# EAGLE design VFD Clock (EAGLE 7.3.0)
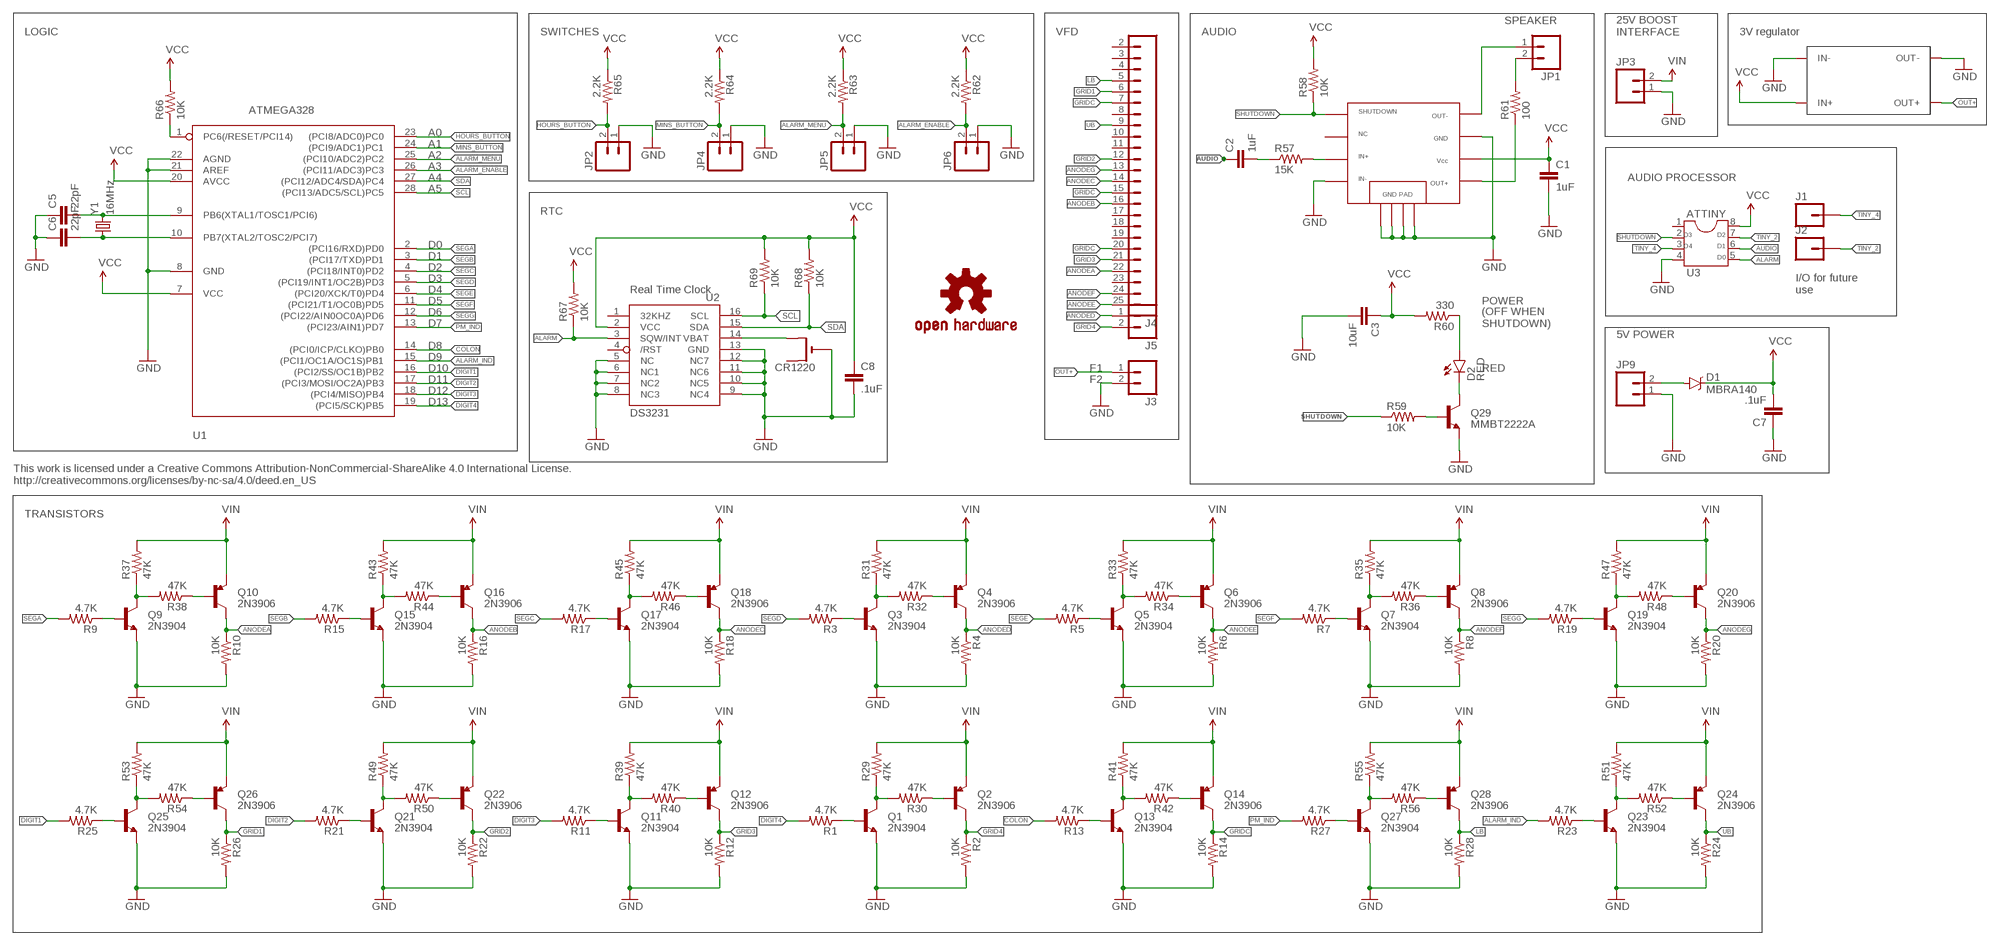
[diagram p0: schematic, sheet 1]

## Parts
ATTINY  U3  DIL8  [DIL08]
C1  1uF  CAPEZ  [CAP-PTH-SMALLEZ]
C2  1uF  CAPEZ  [CAP-PTH-SMALLEZ]
C3  10uF  CAPEZ  [CAP-PTH-SMALLEZ]
C5  22pF  CAPEZ  [CAP-PTH-SMALLEZ]
C6  22pF  CAPEZ  [CAP-PTH-SMALLEZ]
C7  .1uF  CAPEZ  [CAP-PTH-SMALLEZ]
C8  .1uF  CAPEZ  [CAP-PTH-SMALLEZ]
CR1220  CR1220SMT  [CR1220-SMD]
D1  MBRA140  [SMA-DIODE]
D2  RED  LED3MM  [LED3MM]
J1  M01PTH  [1X01]
J2  M01PTH  [1X01]
J3  M02PTH  [1X02]
J4  M24  [1X24]
J5  M02PTH  [1X02]
JP1  M02PTH  [1X02]
JP2  M02PTH  [1X02]
JP3  M02PTH  [1X02]
JP4  M02PTH  [1X02]
JP5  M02PTH  [1X02]
JP6  M02PTH  [1X02]
JP9  M02PTH  [1X02]
Q1  2N3904  TRANSISTOR_NPNTO-92-AMMO  [TO-92-AMMO]
Q2  2N3906  TRANSISTOR_PNPEBC  [TO-92-AMMO]
Q3  2N3904  TRANSISTOR_NPNTO-92-AMMO  [TO-92-AMMO]
Q4  2N3906  TRANSISTOR_PNPEBC  [TO-92-AMMO]
Q5  2N3904  TRANSISTOR_NPNTO-92-AMMO  [TO-92-AMMO]
Q6  2N3906  TRANSISTOR_PNPEBC  [TO-92-AMMO]
Q7  2N3904  TRANSISTOR_NPNTO-92-AMMO  [TO-92-AMMO]
Q8  2N3906  TRANSISTOR_PNPEBC  [TO-92-AMMO]
Q9  2N3904  TRANSISTOR_NPNTO-92-AMMO  [TO-92-AMMO]
Q10  2N3906  TRANSISTOR_PNPEBC  [TO-92-AMMO]
Q11  2N3904  TRANSISTOR_NPNTO-92-AMMO  [TO-92-AMMO]
Q12  2N3906  TRANSISTOR_PNPEBC  [TO-92-AMMO]
Q13  2N3904  TRANSISTOR_NPNTO-92-AMMO  [TO-92-AMMO]
Q14  2N3906  TRANSISTOR_PNPEBC  [TO-92-AMMO]
Q15  2N3904  TRANSISTOR_NPNTO-92-AMMO  [TO-92-AMMO]
Q16  2N3906  TRANSISTOR_PNPEBC  [TO-92-AMMO]
Q17  2N3904  TRANSISTOR_NPNTO-92-AMMO  [TO-92-AMMO]
Q18  2N3906  TRANSISTOR_PNPEBC  [TO-92-AMMO]
Q19  2N3904  TRANSISTOR_NPNTO-92-AMMO  [TO-92-AMMO]
Q20  2N3906  TRANSISTOR_PNPEBC  [TO-92-AMMO]
Q21  2N3904  TRANSISTOR_NPNTO-92-AMMO  [TO-92-AMMO]
Q22  2N3906  TRANSISTOR_PNPEBC  [TO-92-AMMO]
Q23  2N3904  TRANSISTOR_NPNTO-92-AMMO  [TO-92-AMMO]
Q24  2N3906  TRANSISTOR_PNPEBC  [TO-92-AMMO]
Q25  2N3904  TRANSISTOR_NPNTO-92-AMMO  [TO-92-AMMO]
Q26  2N3906  TRANSISTOR_PNPEBC  [TO-92-AMMO]
Q27  2N3904  TRANSISTOR_NPNTO-92-AMMO  [TO-92-AMMO]
Q28  2N3906  TRANSISTOR_PNPEBC  [TO-92-AMMO]
Q29  MMBT2222A  TRANSISTOR_NPNSOT23-3  [SOT23-3]
R1  4.7K  RESISTORPTH-1/4W-VERT  [AXIAL-0.1]
R2  10K  RESISTORPTH-1/4W-VERT  [AXIAL-0.1]
R3  4.7K  RESISTORPTH-1/4W-VERT  [AXIAL-0.1]
R4  10K  RESISTORPTH-1/4W-VERT  [AXIAL-0.1]
R5  4.7K  RESISTORPTH-1/4W-VERT  [AXIAL-0.1]
R6  10K  RESISTORPTH-1/4W-VERT  [AXIAL-0.1]
R7  4.7K  RESISTORPTH-1/4W-VERT  [AXIAL-0.1]
R8  10K  RESISTORPTH-1/4W-VERT  [AXIAL-0.1]
R9  4.7K  RESISTORPTH-1/4W-VERT  [AXIAL-0.1]
R10  10K  RESISTORPTH-1/4W-VERT  [AXIAL-0.1]
R11  4.7K  RESISTORPTH-1/4W-VERT  [AXIAL-0.1]
R12  10K  RESISTORPTH-1/4W-VERT  [AXIAL-0.1]
R13  4.7K  RESISTORPTH-1/4W-VERT  [AXIAL-0.1]
R14  10K  RESISTORPTH-1/4W-VERT  [AXIAL-0.1]
R15  4.7K  RESISTORPTH-1/4W-VERT  [AXIAL-0.1]
R16  10K  RESISTORPTH-1/4W-VERT  [AXIAL-0.1]
R17  4.7K  RESISTORPTH-1/4W-VERT  [AXIAL-0.1]
R18  10K  RESISTORPTH-1/4W-VERT  [AXIAL-0.1]
R19  4.7K  RESISTORPTH-1/4W-VERT  [AXIAL-0.1]
R20  10K  RESISTORPTH-1/4W-VERT  [AXIAL-0.1]
R21  4.7K  RESISTORPTH-1/4W-VERT  [AXIAL-0.1]
R22  10K  RESISTORPTH-1/4W-VERT  [AXIAL-0.1]
R23  4.7K  RESISTORPTH-1/4W-VERT  [AXIAL-0.1]
R24  10K  RESISTORPTH-1/4W-VERT  [AXIAL-0.1]
R25  4.7K  RESISTORPTH-1/4W-VERT  [AXIAL-0.1]
R26  10K  RESISTORPTH-1/4W-VERT  [AXIAL-0.1]
R27  4.7K  RESISTORPTH-1/4W-VERT  [AXIAL-0.1]
R28  10K  RESISTORPTH-1/4W-VERT  [AXIAL-0.1]
R29  47K  RESISTORPTH-1/4W-VERT  [AXIAL-0.1]
R30  47K  RESISTORPTH-1/4W-VERT  [AXIAL-0.1]
R31  47K  RESISTORPTH-1/4W-VERT  [AXIAL-0.1]
R32  47K  RESISTORPTH-1/4W-VERT  [AXIAL-0.1]
R33  47K  RESISTORPTH-1/4W-VERT  [AXIAL-0.1]
R34  47K  RESISTORPTH-1/4W-VERT  [AXIAL-0.1]
R35  47K  RESISTORPTH-1/4W-VERT  [AXIAL-0.1]
R36  47K  RESISTORPTH-1/4W-VERT  [AXIAL-0.1]
R37  47K  RESISTORPTH-1/4W-VERT  [AXIAL-0.1]
R38  47K  RESISTORPTH-1/4W-VERT  [AXIAL-0.1]
R39  47K  RESISTORPTH-1/4W-VERT  [AXIAL-0.1]
R40  47K  RESISTORPTH-1/4W-VERT  [AXIAL-0.1]
R41  47K  RESISTORPTH-1/4W-VERT  [AXIAL-0.1]
R42  47K  RESISTORPTH-1/4W-VERT  [AXIAL-0.1]
R43  47K  RESISTORPTH-1/4W-VERT  [AXIAL-0.1]
R44  47K  RESISTORPTH-1/4W-VERT  [AXIAL-0.1]
R45  47K  RESISTORPTH-1/4W-VERT  [AXIAL-0.1]
R46  47K  RESISTORPTH-1/4W-VERT  [AXIAL-0.1]
R47  47K  RESISTORPTH-1/4W-VERT  [AXIAL-0.1]
R48  47K  RESISTORPTH-1/4W-VERT  [AXIAL-0.1]
R49  47K  RESISTORPTH-1/4W-VERT  [AXIAL-0.1]
R50  47K  RESISTORPTH-1/4W-VERT  [AXIAL-0.1]
R51  47K  RESISTORPTH-1/4W-VERT  [AXIAL-0.1]
R52  47K  RESISTORPTH-1/4W-VERT  [AXIAL-0.1]
R53  47K  RESISTORPTH-1/4W-VERT  [AXIAL-0.1]
R54  47K  RESISTORPTH-1/4W-VERT  [AXIAL-0.1]
R55  47K  RESISTORPTH-1/4W-VERT  [AXIAL-0.1]
R56  47K  RESISTORPTH-1/4W-VERT  [AXIAL-0.1]
R57  15K  RESISTORPTH-1/4W-VERT  [AXIAL-0.1]
R58  10K  RESISTORPTH-1/4W-VERT  [AXIAL-0.1]
R59  10K  RESISTORPTH-1/4W-VERT  [AXIAL-0.1]
R60  330  RESISTORPTH-1/4W-VERT  [AXIAL-0.1]
R61  100  RESISTORPTH-1/4W-VERT  [AXIAL-0.1]
R62  2.2K  RESISTORPTH-1/4W-VERT  [AXIAL-0.1]
R63  2.2K  RESISTORPTH-1/4W-VERT  [AXIAL-0.1]
R64  2.2K  RESISTORPTH-1/4W-VERT  [AXIAL-0.1]
R65  2.2K  RESISTORPTH-1/4W-VERT  [AXIAL-0.1]
R66  10K  RESISTORPTH-1/4W-VERT  [AXIAL-0.1]
R67  10K  RESISTORPTH-1/4W-VERT  [AXIAL-0.1]
R68  10K  RESISTORPTH-1/4W-VERT  [AXIAL-0.1]
R69  10K  RESISTORPTH-1/4W-VERT  [AXIAL-0.1]
U1  ATMEGA328  ATMEGA168PROUND  [DIL28-3-ROUND]
U2  DS3231  DS3231/SO  [SO16W]
U3  TPA2005  [MSOP8]
U$7  OSHW-LOGOS  [OSHW-LOGO-S]
U$10  DCTODC  [DCTODC]
Y1  16MHz  CRYSTALHC49US  [HC49US]

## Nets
ALARM: ATTINY.5 R67.P$1 U2.3(SQW/INT)
ALARM_ENABLE: JP6.2 R62.P$2 U1.26((PCI11/ADC3)PC3)
ALARM_IND: R23.P$2 U1.15((PCI1/OC1A/OC1S)PB1)
ALARM_MENU: JP5.2 R63.P$2 U1.25((PCI10/ADC2)PC2)
ANODEA: J4.22 Q10.3(C) R10.P$1
ANODEB: J4.16 Q16.3(C) R16.P$1
ANODEC: J4.14 Q18.3(C) R18.P$1
ANODED: J5.1 Q4.3(C) R4.P$1
ANODEE: J4.25 Q6.3(C) R6.P$1
ANODEF: J4.24 Q8.3(C) R8.P$1
ANODEG: J4.13 Q20.3(C) R20.P$1
AUDIO: ATTINY.6 C2.1
COLON: R13.P$2 U1.14((PCI0/ICP/CLKO)PB0)
D: Q9.3(C) R37.P$1 R38.P$2
D1: Q15.3(C) R43.P$1 R44.P$2
D2: Q17.3(C) R45.P$1 R46.P$2
D3: Q3.3(C) R31.P$1 R32.P$2
D4: Q5.3(C) R33.P$1 R34.P$2
D5: Q7.3(C) R35.P$1 R36.P$2
D6: Q19.3(C) R47.P$1 R48.P$2
D7: Q25.3(C) R53.P$1 R54.P$2
D8: Q21.3(C) R49.P$1 R50.P$2
D9: Q11.3(C) R39.P$1 R40.P$2
D10: Q1.3(C) R29.P$1 R30.P$2
D11: Q13.3(C) R41.P$1 R42.P$2
D12: Q27.3(C) R55.P$1 R56.P$2
D13: Q23.3(C) R51.P$1 R52.P$2
DIGIT1: R25.P$2 U1.16((PCI2/SS/OC1B)PB2)
DIGIT2: R21.P$2 U1.17((PCI3/MOSI/OC2A)PB3)
DIGIT3: R11.P$2 U1.18((PCI4/MISO)PB4)
DIGIT4: R1.P$2 U1.19((PCI5/SCK)PB5)
GND: ATTINY.4 C1.2 C3.2 C5.1 C6.1 C7.1 C8.2 CR1220.- J3.2 JP2.1 JP3.1 JP4.1 JP5.1 JP6.1 JP9.1 Q1.1(E) Q3.1(E) Q5.1(E) Q7.1(E) Q9.1(E) Q11.1(E) Q13.1(E) Q15.1(E) Q17.1(E) Q19.1(E) Q21.1(E) Q23.1(E) Q25.1(E) Q27.1(E) Q29.2(E) R2.P$2 R4.P$2 R6.P$2 R8.P$2 R10.P$2 R12.P$2 R14.P$2 R16.P$2 R18.P$2 R20.P$2 R22.P$2 R24.P$2 R26.P$2 R28.P$2 U1.8(GND) U1.21(AREF) U1.22(AGND) U2.5(NC) U2.6(NC1) U2.7(NC2) U2.8(NC3) U2.9(NC4) U2.10(NC5) U2.11(NC6) U2.12(NC7) U2.13(GND) U3.4 U3.7 U3.A U3.B U3.C U3.D U$10.IN- U$10.OUT-
GRID1: J4.6 Q26.3(C) R26.P$1
GRID2: J4.12 Q22.3(C) R22.P$1
GRID3: J4.21 Q12.3(C) R12.P$1
GRID4: J5.2 Q2.3(C) R2.P$1
GRIDC: J4.7 J4.15 J4.20 Q14.3(C) R14.P$1
HOURS_BUTTON: JP2.2 R65.P$2 U1.23((PCI8/ADC0)PC0)
IN+AMP: R57.P$2 U3.3
LB: J4.5 Q28.3(C) R28.P$1
MINS_BUTTON: JP4.2 R64.P$2 U1.24((PCI9/ADC1)PC1)
N$1: Q15.2(B) R15.P$1
N$2: Q16.2(B) R44.P$1
N$3: Q17.2(B) R17.P$1
N$4: Q18.2(B) R46.P$1
N$5: Q3.2(B) R3.P$1
N$6: Q4.2(B) R32.P$1
N$7: CR1220.+$2(+1) U2.14(VBAT)
N$8: Q5.2(B) R5.P$1
N$9: Q6.2(B) R34.P$1
N$10: Q9.2(B) R9.P$1
N$11: Q7.2(B) R7.P$1
N$12: Q8.2(B) R36.P$1
N$13: Q10.2(B) R38.P$1
N$14: Q19.2(B) R19.P$1
N$15: Q20.2(B) R48.P$1
N$16: Q25.2(B) R25.P$1
N$17: Q26.2(B) R54.P$1
N$18: Q21.2(B) R21.P$1
N$19: Q22.2(B) R50.P$1
N$20: Q11.2(B) R11.P$1
N$21: Q12.2(B) R40.P$1
N$22: Q1.2(B) R1.P$1
N$23: Q2.2(B) R30.P$1
N$24: Q13.2(B) R13.P$1
N$25: Q14.2(B) R42.P$1
N$26: Q27.2(B) R27.P$1
N$27: Q28.2(B) R56.P$1
N$28: JP1.2 R61.P$2
N$29: D2.A R60.P$1
N$30: Q23.2(B) R23.P$1
N$31: Q29.1(B) R59.P$2
N$32: Q24.2(B) R52.P$1
N$33: D2.K(C) Q29.3(C)
N$34: C2.2 R57.P$1
N$35: JP1.1 U3.8
N$36: R61.P$1 U3.5
N$37: C5.2 U1.9(PB6(XTAL1/TOSC1/PCI6)) Y1.2
N$38: C6.2 U1.10(PB7(XTAL2/TOSC2/PCI7)) Y1.1
N$39: D1.A JP9.2
OUT+: J3.1 U$10.OUT+
PM_IND: R27.P$2 U1.13((PCI23/AIN1)PD7)
RESET: R66.P$1 U1.1(PC6(/RESET/PCI14))
SCL: R69.P$1 U1.28((PCI13/ADC5/SCL)PC5) U2.16(SCL)
SDA: R68.P$1 U1.27((PCI12/ADC4/SDA)PC4) U2.15(SDA)
SEGA: R9.P$2 U1.2((PCI16/RXD)PD0)
SEGB: R15.P$2 U1.3((PCI17/TXD)PD1)
SEGC: R17.P$2 U1.4((PCI18/INT0)PD2)
SEGD: R3.P$2 U1.5((PCI19/INT1/OC2B)PD3)
SEGE: R5.P$2 U1.6((PCI20/XCK/T0)PD4)
SEGF: R7.P$2 U1.11((PCI21/T1/OC0B)PD5)
SEGG: R19.P$2 U1.12((PCI22/AIN0OC0A)PD6)
SHUTDOWN: ATTINY.2 R58.P$1 R59.P$1 U3.1
TINY_2: ATTINY.7 J2.1
TINY_4: ATTINY.3 J1.1
UB: J4.9 Q24.3(C) R24.P$1
VCC: ATTINY.8 C1.1 C3.1 C7.2 C8.1 D1.C R58.P$2 R60.P$2 R62.P$1 R63.P$1 R64.P$1 R65.P$1 R66.P$2 R67.P$2 R68.P$2 R69.P$2 U1.7(VCC) U1.20(AVCC) U2.2(VCC) U3.6 U$10.IN+
VIN: JP3.2 Q2.1(E) Q4.1(E) Q6.1(E) Q8.1(E) Q10.1(E) Q12.1(E) Q14.1(E) Q16.1(E) Q18.1(E) Q20.1(E) Q22.1(E) Q24.1(E) Q26.1(E) Q28.1(E) R29.P$2 R31.P$2 R33.P$2 R35.P$2 R37.P$2 R39.P$2 R41.P$2 R43.P$2 R45.P$2 R47.P$2 R49.P$2 R51.P$2 R53.P$2 R55.P$2
Unconnected: ATTINY.1 CR1220.+$1(+) J4.2 J4.3 J4.4 J4.8 J4.10 J4.11 J4.17 J4.18 J4.19 J4.23 U2.1(32KHZ) U2.4(/RST) U3.NC

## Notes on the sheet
- SPEAKER
- LOGIC | SWITCHES | VFD | AUDIO
- 25V BOOST
  INTERFACE
- 3V regulator
- A0
- A1
- A2
- A3
- A4 | AUDIO PROCESSOR
- A5
- RTC
- D3 | D2
- D0 | D4 | D1
- D1 | D0
- D2
- D3
- D4 | Real Time Clock
- I/O for future
  use
- D5 | POWER
- D6
- D7
- (OFF WHEN 
  SHUTDOWN)
- 5V POWER
- D8
- D9
- D10 | F1 | RED
- D11 | F2
- D12
- D13
- This work is licensed under a Creative Commons Attribution-NonCommercial-ShareAlike 4.0 International License.
  http://creativecommons.org/licenses/by-nc-sa/4.0/deed.en_US
- TRANSISTORS

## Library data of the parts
ATTINY = ic-package:DIL8: Dual In Line / Socket
C1-C3 C5-C8 = SparkFun-Capacitors:CAP: Capacitor
CR1220 = adafruit:CR1220: CR1216/CR1220/CR1225 12mm 3V lithium coin cell Great for battery packup. Both SMT and THM holders. Note the THM package has the ground pads on both sides of the PCB so that the masks are the same - this reduces the cost
D1 = SparkFun-DiscreteSemi:MBRA140: 40V, 1A Schottky rectifier; PROD_ID: DIO-08053
D2 = SparkFun-LED:LED: LEDs; PROD_ID: DIO-08794
J1 J2 = SparkFun-Connectors:M01: Header 1
J3 J5 = SparkFun-Connectors:M02: Standard 2-pin 0.1" header. Use with
J4 = SparkFun-Connectors:M24: 1x24 .1" header
JP1-JP6 JP9 = SparkFun:M02: Header 2
Q1 Q3 Q5 Q7 Q9 Q11 Q13 Q15 Q17 Q19 Q21 Q23 Q25 Q27 = SparkFun-DiscreteSemi:TRANSISTOR_NPN: Generic NPN BJT MMBT2222A - TRANS-08049 (SOT-23, 1A 40V) MPSA42 - TRANS-09116 (SOT-23, 500mA 300V) MMBT5088LT1G - TRANS-11160 (SOT-23, 50 mA 30V)
Q2 Q4 Q6 Q8 Q10 Q12 Q14 Q16 Q18 Q20 Q22 Q24 Q26 Q28 = SparkFun-DiscreteSemi:TRANSISTOR_PNP: Generic PNP BJT Double check pinouts against datasheets- not all devices are the same! MMBT3906 - 40V 200mA SOT-23 (TRANS-08052) MMBT4403 - 40V 600mA SOT-23 (TRANS-09245)
Q29 = SparkFun:TRANSISTOR_NPN: Transistor NPN BJT configuration in SOT23 package. MMBT2222 is the common NPN we use. Double check BCE configuration again layout.
R1-R69 = SparkFun-Resistors:RESISTOR: Resistor
U1 = adafruit:ATMEGA168*P: MICROCONTROLLER 16 kBytes FLASH 1 kBytes SRAM 512 Bytes EEPROM USART 8-channel 10 bit ADC
U2 = adafruit:DS3231
U3 = TPA2005:TPA2005
U$7 = SparkFun:OSHW-LOGO: Open Source Hardware Logo This logo indicates the piece of hardware it is found on incorporates a OSHW license and/or adheres to the definition of open source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
U$10 = DC to DC:DCTODC
Y1 = SparkFun-FreqCtrl:CRYSTAL: Various standard crystals. Proven footprints.

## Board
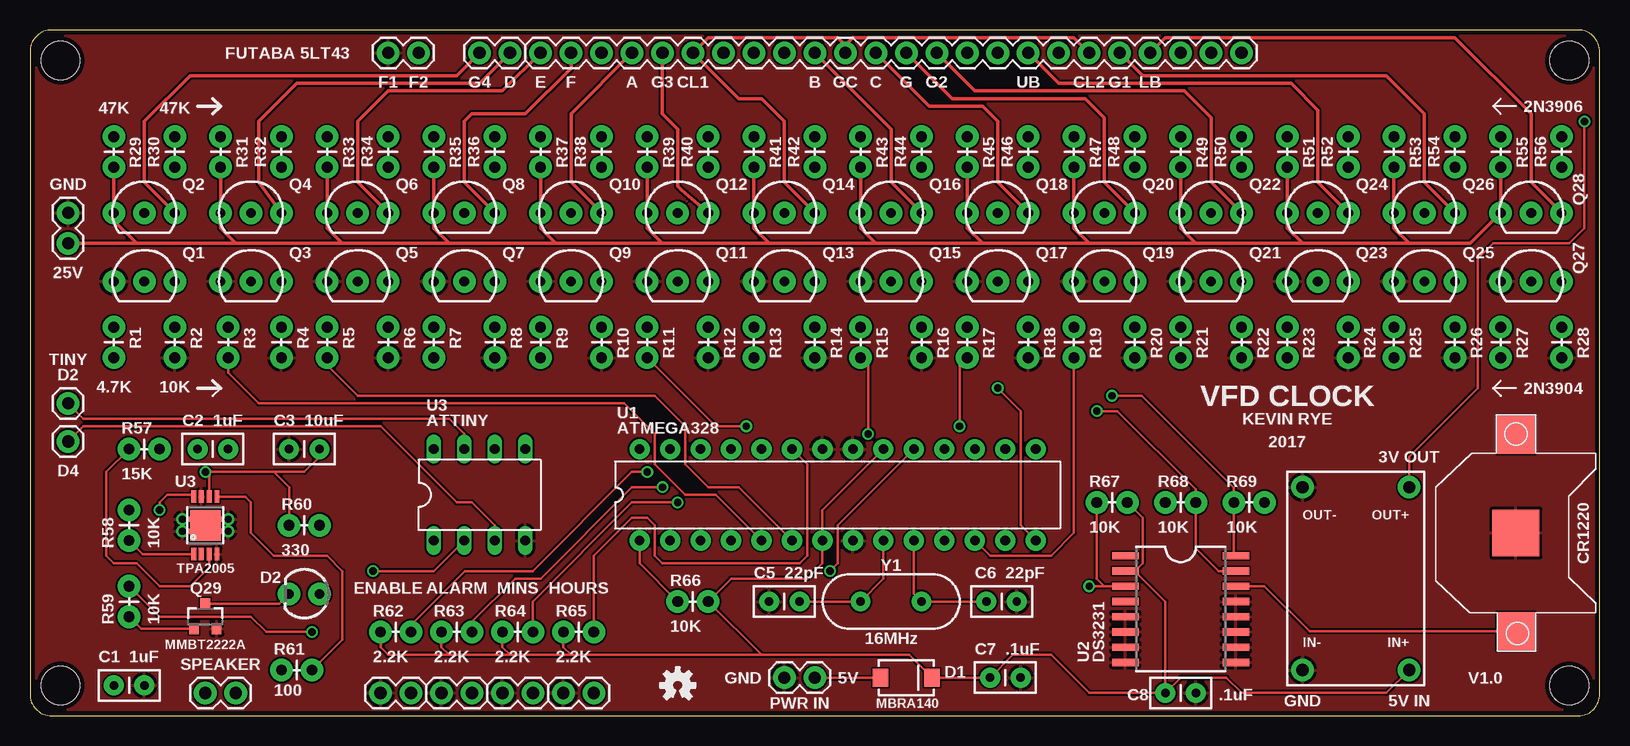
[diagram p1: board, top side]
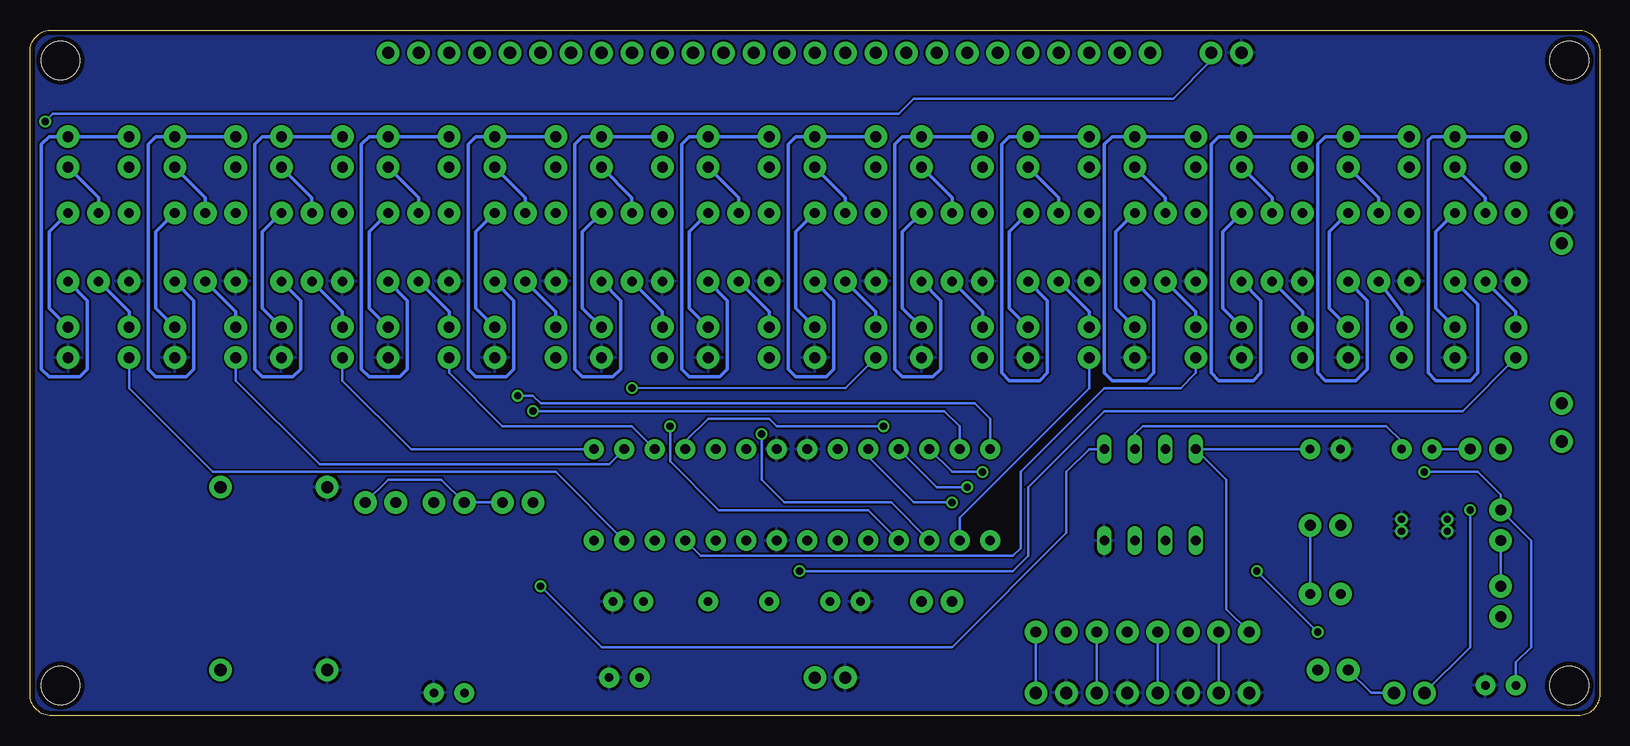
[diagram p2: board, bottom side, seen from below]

Size 130.81 x 57.15 mm. Coordinates in mm from the lower left corner, seen from the top.
Outline: 0,55.35 0,1.8 arc90 1.8,0 129.01,0 arc90 130.81,1.8 130.81,55.35 arc90 129.01,57.15 1.8,57.15 arc90 0,55.35
Copper layers (1*16): Top 0.0356mm / dielectric 1.5011mm / Bottom 0.0356mm
Design rules "oshpark-2layer": minimum track width 6mil, minimum drill 13mil, track to track 6mil, track to pad 6mil, pad to pad 6mil, via to via 6mil, smd to smd 6mil, copper to edge 15mil, drill to drill 6mil, minimum pad ring 7mil, minimum via ring 7mil, stop-mask expansion 2.5mil, vias tented up to drill 0mil, thermal gap 10mil
Holes 3.2 mm at 2.54,54.61 128.27,54.61 128.27,2.54 2.54,2.54

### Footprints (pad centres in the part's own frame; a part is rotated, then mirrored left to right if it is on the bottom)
DIL08 = drill 0.813 long: 1 -3.81,-3.81; 2 -1.27,-3.81; 3 1.27,-3.81; 4 3.81,-3.81; 5 3.81,3.81; 6 1.27,3.81; 7 -1.27,3.81; 8 -3.81,3.81
CAP-PTH-SMALLEZ = drill 0.7 pad 1.651: 1 0,0; 2 2.54,0
CR1220-SMD = smd 3.2 x 3.2: +$1 -8.2,0; +$2 8.2,0 | smd 3.9 x 3.9: - 0,0
SMA-DIODE = smd 1.27 x 1.47: A -2.15,0; C 2.15,0
LED3MM = drill 0.813 pad 1.88: A -1.27,0; K 1.27,0
1X01 = drill 1.016 pad 1.88: 1 0,0
1X02 = drill 1.016 pad 1.88: 1 0,0; 2 2.54,0
1X24 = drill 1.016 pad 1.88: 2 -26.67,0; 3 -24.13,0; 4 -21.59,0; 5 -19.05,0; 6 -16.51,0; 7 -13.97,0; 8 -11.43,0; 9 -8.89,0; 10 -6.35,0; 11 -3.81,0; 12 -1.27,0; 13 1.27,0; 14 3.81,0; 15 6.35,0; 16 8.89,0; 17 11.43,0; 18 13.97,0; 19 16.51,0; 20 19.05,0; 21 21.59,0; 22 24.13,0; 23 26.67,0; 24 29.21,0; 25 31.75,0
TO-92-AMMO = drill 0.813 pad 1.88: 1 -2.54,0; 2 0,0; 3 2.54,0
SOT23-3 = smd 0.8 x 0.9: 1 -0.95,-1; 2 0.95,-1; 3 0,1.1
AXIAL-0.1 = drill 0.9 pad 1.88: P$1 0,0; P$2 2.54,0
DIL28-3-ROUND = drill 0.813 pad 1.676: 1 -16.51,-3.81; 2 -13.97,-3.81; 3 -11.43,-3.81; 4 -8.89,-3.81; 5 -6.35,-3.81; 6 -3.81,-3.81; 7 -1.27,-3.81; 8 1.27,-3.81; 9 3.81,-3.81; 10 6.35,-3.81; 11 8.89,-3.81; 12 11.43,-3.81; 13 13.97,-3.81; 14 16.51,-3.81; 15 16.51,3.81; 16 13.97,3.81; 17 11.43,3.81; 18 8.89,3.81; 19 6.35,3.81; 20 3.81,3.81; 21 1.27,3.81; 22 -1.27,3.81; 23 -3.81,3.81; 24 -6.35,3.81; 25 -8.89,3.81; 26 -11.43,3.81; 27 -13.97,3.81; 28 -16.51,3.81
SO16W = smd 0.6 x 2.2: 1 -4.445,-4.6; 2 -3.175,-4.6; 3 -1.905,-4.6; 4 -0.635,-4.6; 5 0.635,-4.6; 6 1.905,-4.6; 7 3.175,-4.6; 8 4.445,-4.6; 9 4.445,4.6; 10 3.175,4.6; 11 1.905,4.6; 12 0.635,4.6; 13 -0.635,4.6; 14 -1.905,4.6; 15 -3.175,4.6; 16 -4.445,4.6
MSOP8 = smd 0.41 x 1.02: 1 -0.975,-2.4; 3 0.325,-2.4; 4 0.975,-2.4; 5 0.975,2.4; 6 0.325,2.4; 7 -0.325,2.4; 8 -0.975,2.4; NC -0.325,-2.4 | smd 1.02 x 0.41: 2 -1.13,0.5; 9 -1.13,-0.5; 10 1.13,-0.5; 11 1.13,0.5 | drill 0.61 pad 1.016: A -1.9,-0.5; B 1.91,-0.5; C 1.91,0.5; D -1.9,0.5 | smd 2.54 x 1.27: GND 0,0.635; GND1 0,0.635; GND* 0,-0.635
DCTODC = drill 1.016 pad 1.88: IN+ 10.16,1.27; IN- 1.27,1.27; OUT+ 10.16,16.51; OUT- 1.27,16.51
HC49US = drill 0.7 pad 1.651: 1 -2.54,0; 2 2.54,0

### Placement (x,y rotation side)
ATTINY  37.47,18.41 0 top
C1  6.99,2.54 0 top
C2  16.51,22.23 180 top
C3  24.13,22.23 180 top
C5  61.59,9.53 0 top
C6  82.23,9.53 180 top
C7  82.55,3.18 180 top
C8  94.61,1.91 0 top
CR1220  123.82,15.24 270 top
D1  73.02,3.18 0 top
D2  22.86,10.16 180 top
J1  3.17,22.86 0 top
J2  3.17,26.04 0 top
J3  32.39,55.24 180 top
J4  74.3,55.24 180 top
J5  40.01,55.24 180 top
JP1  14.61,1.91 0 top
JP2  44.45,1.91 0 top
JP3  3.17,41.91 270 top
JP4  39.37,1.91 0 top
JP5  34.29,1.91 0 top
JP6  29.21,1.91 0 top
JP9  62.87,3.18 0 top
Q1  9.53,36.2 0 top
Q2  9.53,41.91 0 top
Q3  18.41,36.2 0 top
Q4  18.41,41.91 0 top
Q5  27.3,36.2 0 top
Q6  27.3,41.91 0 top
Q7  36.2,36.2 0 top
Q8  36.2,41.91 0 top
Q9  45.09,36.2 0 top
Q10  45.09,41.91 0 top
Q11  53.98,36.2 0 top
Q12  53.98,41.91 0 top
Q13  62.87,36.2 0 top
Q14  62.87,41.91 0 top
Q15  71.75,36.2 0 top
Q16  71.75,41.91 0 top
Q17  80.64,36.2 0 top
Q18  80.64,41.91 0 top
Q19  89.53,36.2 0 top
Q20  89.53,41.91 0 top
Q21  98.42,36.2 0 top
Q22  98.42,41.91 0 top
Q23  107.31,36.2 0 top
Q24  107.31,41.91 0 top
Q25  116.2,36.2 0 top
Q26  116.2,41.91 0 top
Q27  125.09,36.2 0 top
Q28  125.09,41.91 0 top
Q29  14.61,8.26 0 top
R1  6.99,32.38 270 top
R2  12.06,32.38 270 top
R3  16.51,32.38 270 top
R4  20.95,32.38 270 top
R5  24.76,32.38 270 top
R6  29.84,32.38 270 top
R7  33.66,32.38 270 top
R8  38.73,32.38 270 top
R9  42.55,32.38 270 top
R10  47.62,32.38 270 top
R11  51.44,32.38 270 top
R12  56.52,32.38 270 top
R13  60.33,32.38 270 top
R14  65.41,32.38 270 top
R15  69.21,32.38 270 top
R16  74.3,32.38 270 top
R17  78.1,32.38 270 top
R18  83.18,32.38 270 top
R19  86.99,32.38 270 top
R20  92.07,32.38 270 top
R21  95.88,32.38 270 top
R22  100.96,32.38 270 top
R23  104.77,32.38 270 top
R24  109.85,32.38 270 top
R25  113.66,32.38 270 top
R26  118.74,32.38 270 top
R27  122.55,32.38 270 top
R28  127.64,32.38 270 top
R29  6.99,48.26 270 top
R30  12.06,45.72 90 top
R31  15.88,48.26 270 top
R32  20.95,45.72 90 top
R33  24.76,48.26 270 top
R34  29.84,45.72 90 top
R35  33.66,48.26 270 top
R36  38.73,45.72 90 top
R37  42.55,48.26 270 top
R38  47.62,45.72 90 top
R39  51.44,48.26 270 top
R40  56.52,45.72 90 top
R41  60.33,48.26 270 top
R42  65.41,45.72 90 top
R43  69.21,48.26 270 top
R44  74.3,45.72 90 top
R45  78.1,48.26 270 top
R46  83.18,45.72 90 top
R47  86.99,48.26 270 top
R48  92.07,45.72 90 top
R49  95.88,48.26 270 top
R50  100.96,45.72 90 top
R51  104.77,48.26 270 top
R52  109.85,45.72 90 top
R53  113.66,48.26 270 top
R54  118.74,45.72 90 top
R55  122.55,48.26 270 top
R56  127.64,45.72 90 top
R57  10.79,22.23 180 top
R58  8.26,14.61 90 top
R59  8.26,10.8 270 top
R60  24.13,15.88 180 top
R61  23.49,3.81 180 top
R62  29.21,6.98 0 top
R63  34.29,6.98 0 top
R64  39.37,6.98 0 top
R65  44.45,6.98 0 top
R66  53.98,9.53 0 top
R67  88.9,17.78 0 top
R68  97.16,17.78 180 top
R69  100.33,17.78 0 top
U1  67.31,18.41 0 top
U2  95.88,8.89 270 top
U3  14.61,15.88 0 top
U$7  53.98,2.54 0 top
U$10  104.77,2.54 0 top
Y1  71.75,9.53 180 top

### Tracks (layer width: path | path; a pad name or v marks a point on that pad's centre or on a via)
ALARM  (via drill 0.61)
  Top 0.203: U2.3 89.53,10.8 | 89.53,10.8 88.9,11.43 R67.P$1 | v88.27,10.8 89.53,10.8
  Bottom 0.203: ATTINY.5 42.55,22.23 44.45,20.32 44.45,15.24 53.98,5.71 83.18,5.71 v88.27,10.8
ALARM_ENABLE  (via drill 0.61)
  Top 0.203: v51.44,20.32 50.16,20.32 41.91,12.07 36.24,12.07 31.75,7.57 R62.P$2
  Bottom 0.203: JP6.2 R62.P$2 | U1.26 53.98,20.32 v51.44,20.32
ALARM_IND
  Bottom 0.203: U1.15 99.06,22.23 104.77,27.94 R23.P$2
ALARM_MENU  (via drill 0.61)
  Top 0.203: v52.71,19.05 50.16,19.05 42.55,11.43 40.42,11.43 36.83,7.84 R63.P$2
  Bottom 0.203: JP5.2 R63.P$2 | U1.25 55.25,19.05 v52.71,19.05
ANODEA
  Top 0.305: Q10.3 45.09,44.45 45.09,50.16 J4.22
  Bottom 0.305: Q10.3 49.21,40.32 49.21,33.97 R10.P$1
ANODEB
  Top 0.305: Q16.3 71.75,44.45 71.75,48.9 J4.16
  Bottom 0.305: R16.P$1 75.88,33.97 75.88,40.32 Q16.3
ANODEC
  Top 0.305: Q18.3 80.64,44.45 80.64,49.53 79.38,50.8 74.93,50.8 J4.14
  Bottom 0.305: R18.P$1 84.77,33.97 84.77,40.32 Q18.3
ANODED
  Top 0.305: Q4.3 19.05,44.45 19.05,49.53 22.22,52.71 37.47,52.71 J5.1
  Bottom 0.305: R4.P$1 22.54,33.97 22.54,40.32 Q4.3
ANODEE
  Top 0.305: Q6.3 27.3,44.45 27.3,49.53 29.84,52.07 39.37,52.07 J4.25
  Bottom 0.305: R6.P$1 31.43,33.97 31.43,40.32 Q6.3
ANODEF
  Top 0.305: Q8.3 36.2,44.45 36.2,49.53 36.83,50.16 41.27,50.16 45.09,53.98 J4.24
  Bottom 0.305: R8.P$1 40.32,33.97 40.32,40.32 Q8.3
ANODEG
  Top 0.305: Q20.3 89.53,44.45 89.53,49.85 87.95,51.43 76.83,51.43 J4.13
  Bottom 0.305: R20.P$1 93.66,33.97 93.66,40.32 Q20.3
AUDIO
  Bottom 0.203: C2.1 16.51,22.86 17.78,24.13 38.1,24.13 38.73,23.49 ATTINY.6
COLON  (via drill 0.61)
  Top 0.203: U1.14 82.55,15.88 82.55,25.4 v80.64,27.3
  Bottom 0.178: 62.87,27.3 v80.64,27.3
  Bottom 0.203: R13.P$2 62.87,27.3
D
  Bottom 0.305: R37.P$1 R38.P$2 49.21,48.26 49.85,47.63 49.85,28.58 49.21,27.94 46.67,27.94 46.04,28.58 46.04,34.61 Q9.3
D1
  Bottom 0.305: R43.P$1 R44.P$2 75.88,48.26 76.52,47.63 76.52,28.89 75.88,28.26 73.34,28.26 72.71,28.89 72.71,34.61 Q15.3
D2
  Bottom 0.305: R45.P$1 R46.P$2 84.77,48.26 85.41,47.63 85.41,28.89 84.77,28.26 82.23,28.26 81.6,28.89 81.6,34.61 Q17.3
D3
  Bottom 0.305: R31.P$1 R32.P$2 22.86,48.26 23.49,47.63 23.49,28.58 22.86,27.94 20.32,27.94 19.37,28.89 19.37,34.61 Q3.3
D4
  Bottom 0.305: R33.P$1 R34.P$2 31.75,48.26 32.39,47.63 32.39,28.58 31.75,27.94 28.89,27.94 28.26,28.58 28.26,34.61 Q5.3
D5
  Bottom 0.305: R35.P$1 R36.P$2 40.64,48.26 41.27,47.63 41.27,28.58 40.64,27.94 37.78,27.94 37.15,28.58 37.15,34.61 Q7.3
D6
  Bottom 0.305: R47.P$1 R48.P$2 93.66,48.26 94.3,47.63 94.3,28.89 93.66,28.26 91.12,28.26 90.49,28.89 90.49,34.61 Q19.3
D7
  Bottom 0.305: R53.P$1 R54.P$2 120.33,48.26 120.97,47.63 120.97,28.89 120.33,28.26 117.79,28.26 117.16,28.89 117.16,34.61 Q25.3
D8
  Bottom 0.305: R49.P$1 R50.P$2 102.55,48.26 103.19,47.63 103.19,28.89 102.55,28.26 100.01,28.26 99.38,28.89 99.38,34.61 Q21.3
D9
  Bottom 0.305: R39.P$1 R40.P$2 58.1,48.26 58.74,47.63 58.74,28.89 58.1,28.26 55.56,28.26 54.93,28.89 54.93,34.61 Q11.3
D10
  Bottom 0.305: R29.P$1 R30.P$2 13.97,48.26 14.29,47.94 14.29,28.58 13.65,27.94 10.79,27.94 10.16,28.58 10.16,34.29 Q1.3
D11
  Bottom 0.305: R41.P$1 R42.P$2 66.99,48.26 67.63,47.63 67.63,28.89 66.99,28.26 64.45,28.26 63.82,28.89 63.82,34.61 Q13.3
D12
  Bottom 0.305: R55.P$1 R56.P$2 129.22,48.26 129.86,47.63 129.86,28.89 129.22,28.26 126.68,28.26 126.05,28.89 126.05,34.61 Q27.3
D13
  Bottom 0.305: R51.P$1 R52.P$2 111.44,48.26 112.08,47.63 112.08,28.89 111.44,28.26 108.9,28.26 108.27,28.89 108.27,34.61 Q23.3
DIGIT1
  Bottom 0.203: U1.16 82.55,20.95 106.68,20.95 113.66,27.94 R25.P$2
DIGIT2
  Bottom 0.203: R21.P$2 95.88,28.58 91.44,24.13 80.64,24.13 U1.17
DIGIT3  (via drill 0.61)
  Top 0.203: v59.69,24.13 57.15,24.13 R11.P$2
  Bottom 0.203: U1.18 76.2,22.86 74.3,24.77 69.21,24.77 68.58,24.13 v59.69,24.13
DIGIT4  (via drill 0.61)
  Top 0.203: v66.67,12.07 67.31,12.7 67.31,15.88 U1.19
  Bottom 0.203: R1.P$2 11.43,25.4 41.27,25.4 47.62,19.05 47.62,13.34 48.9,12.07 v66.67,12.07
GND
  pour Bottom: -0.64,57.79 131.45,57.79 131.45,-0.63 -0.64,-0.63
  pour Top: -1.27,58.42 132.4,58.42 132.4,-1.27 -1.27,-1.27
GRID1
  Top 0.305: Q26.3 116.2,44.45 116.2,50.16 113.03,53.34 92.71,53.34 J4.6
  Bottom 0.305: R26.P$1 120.33,33.97 120.33,40.32 Q26.3
GRID2
  Top 0.305: Q22.3 98.42,44.45 98.42,49.85 96.2,52.07 78.74,52.07 J4.12
  Bottom 0.305: R22.P$1 102.55,33.97 102.55,40.32 Q22.3
GRID3
  Top 0.305: Q12.3 54.29,43.81 53.98,44.13 53.98,48.9 52.71,50.16 J4.21
  Bottom 0.305: Q12.3 58.1,40.32 58.1,33.97 R12.P$1
GRID4
  Top 0.305: Q2.3 9.53,44.45 9.53,49.53 13.34,53.34 35.56,53.34 J5.2
  Bottom 0.305: R2.P$1 13.65,33.97 13.65,40.32 Q2.3
GRIDC
  Top 0.305: Q14.3 62.87,44.45 62.87,49.53 60.96,51.43 59.05,51.43 J4.20 56.52,56.52 67.31,56.52 67.94,55.88 | J4.15 67.94,55.88 | 67.94,55.88 68.58,56.52 86.99,56.52 J4.7
  Bottom 0.305: R14.P$1 66.99,33.97 66.99,40.32 Q14.3
HOURS_BUTTON
  Top 0.203: U1.23 64.77,20.95 64.77,13.34 64.13,12.7 52.71,12.7 52.07,13.34 52.07,15.88 51.44,16.51 50.16,16.51 46.99,13.34 R65.P$2
  Bottom 0.203: JP2.2 R65.P$2
IN+AMP
  Top 0.203: U3.3 14.93,12.39 13.34,10.8 10.79,10.8 8.89,12.7 6.99,12.7 6.35,13.34 6.35,20.32 R57.P$2
LB
  Top 0.305: Q28.3 125.09,44.45 125.09,50.16 118.74,56.52 94.61,56.52 J4.5
  Bottom 0.305: R28.P$1 129.22,33.97 129.22,40.32 Q28.3
MINS_BUTTON  (via drill 0.61)
  Top 0.203: v53.98,17.78 50.16,17.78 41.91,9.53 R64.P$2
  Bottom 0.203: JP4.2 R64.P$2 | U1.24 60.96,21.59 57.15,17.78 v53.98,17.78
N$1
  Bottom 0.305: R15.P$1 69.21,33.66 Q15.2
N$2
  Bottom 0.305: Q16.2 71.75,43.18 R44.P$1
N$3
  Bottom 0.305: R17.P$1 78.1,33.66 Q17.2
N$4
  Bottom 0.305: Q18.2 80.64,43.18 R46.P$1
N$5
  Bottom 0.305: R3.P$1 16.51,33.66 Q3.2
N$6
  Bottom 0.305: Q4.2 18.41,43.18 R32.P$1
N$7
  Top 0.203: CR1220.+$2 106.62,7.04 102.87,10.8 U2.14
N$8
  Bottom 0.305: R5.P$1 24.76,33.66 Q5.2
N$9
  Bottom 0.305: Q6.2 27.3,43.18 R34.P$1
N$10
  Bottom 0.305: R9.P$1 42.55,33.66 Q9.2
N$11
  Bottom 0.305: R7.P$1 33.66,33.66 Q7.2
N$12
  Bottom 0.305: Q8.2 36.2,43.18 R36.P$1
N$13
  Bottom 0.305: Q10.2 45.09,43.18 R38.P$1
N$14
  Bottom 0.305: R19.P$1 86.99,33.66 Q19.2
N$15
  Bottom 0.305: Q20.2 89.53,43.18 R48.P$1
N$16
  Bottom 0.305: R25.P$1 113.66,33.66 Q25.2
N$17
  Bottom 0.305: Q26.2 116.2,43.18 R54.P$1
N$18
  Bottom 0.305: R21.P$1 95.88,33.66 Q21.2
N$19
  Bottom 0.305: Q22.2 98.42,43.18 R50.P$1
N$20
  Bottom 0.305: R11.P$1 51.44,33.66 Q11.2
N$21
  Bottom 0.305: Q12.2 53.98,43.18 R40.P$1
N$22
  Bottom 0.305: R1.P$1 6.99,33.66 Q1.2
N$23
  Bottom 0.305: Q2.2 9.53,43.18 R30.P$1
N$24
  Bottom 0.305: R13.P$1 60.33,33.66 Q13.2
N$25
  Bottom 0.305: Q14.2 62.87,43.18 R42.P$1
N$26
  Bottom 0.305: R27.P$1 122.55,33.66 Q27.2
N$27
  Bottom 0.305: Q28.2 125.09,43.18 R56.P$1
N$28
  Bottom 0.203: JP1.2 19.05,1.91 R61.P$2
N$29
  Bottom 0.203: R60.P$1 D2.A
N$30
  Bottom 0.305: R23.P$1 104.77,33.66 Q23.2
N$31
  Top 0.203: Q29.1 9.26,7.26 R59.P$2
N$32
  Bottom 0.305: Q24.2 107.31,43.18 R52.P$1
N$33
  Top 0.203: Q29.3 20.79,9.36 D2.K
N$34
  Bottom 0.203: R57.P$1 C2.2
N$35  (via drill 0.61)
  Top 0.203: v10.79,17.15 10.79,17.78 11.43,18.41 13.49,18.41 U3.8
  Bottom 0.203: JP1.1 10.79,5.71 v10.79,17.15
N$36
  Top 0.203: U3.5 17.92,18.27 18.41,17.78 18.41,15.24 20.32,13.34 24.76,13.34 26.04,12.07 26.04,6.35 R61.P$1
N$37
  Top 0.203: C5.2 Y1.2 71.12,11.43 U1.9
N$38
  Top 0.203: C6.2 Y1.1 73.66,10.16 U1.10
N$39
  Top 0.203: JP9.2 D1.A
OUT+  (via drill 0.61)
  Top 0.203: v129.54,49.53 129.54,40.64 128.27,39.37 121.92,39.37 120.65,38.1 120.65,27.3 114.93,21.59 U$10.OUT+
  Bottom 0.203: J3.1 32.39,54.61 35.56,51.43 57.15,51.43 58.42,50.16 128.91,50.16 v129.54,49.53
PM_IND
  Bottom 0.203: U1.13 86.99,20.32 115.57,20.32 122.55,27.3 R27.P$2
RESET
  Top 0.203: R66.P$1 50.8,12.7 U1.1
SCL  (via drill 0.61)
  Top 0.203: U2.16 100.33,13.65 R69.P$1 100.33,19 92.66,26.67 v90.17,26.67
  Bottom 0.203: U1.28 50.8,24.77 52.07,26.04 88.27,26.04 88.9,26.67 v90.17,26.67
SDA  (via drill 0.61)
  Top 0.203: U2.15 99.06,12.07 97.16,13.97 R68.P$1 97.16,18.86 90.62,25.4 v88.9,25.4
  Bottom 0.203: U1.27 53.34,24.13 54.61,25.4 v88.9,25.4
SEGA
  Bottom 0.203: U1.2 53.34,16.51 42.55,27.3 R9.P$2
SEGB  (via drill 0.61)
  Top 0.203: R15.P$2 69.85,29.21 v69.85,23.49
  Bottom 0.203: v69.85,23.49 69.85,19.69 67.94,17.78 59.05,17.78 U1.3
SEGC  (via drill 0.61)
  Top 0.203: R17.P$2 77.47,29.21 v77.47,24.13
  Bottom 0.203: v77.47,24.13 77.47,21.21 73.4,17.15 60.96,17.15 U1.4
SEGD
  Top 0.203: R3.P$2 16.51,28.58 19.05,26.04 49.53,26.04 52.07,23.49 52.07,20.95 54.61,18.41 57.15,18.41 U1.5
SEGE
  Top 0.203: R5.P$2 24.76,29.21 27.3,26.67 52.07,26.67 54.61,24.13 54.61,20.95 56.52,19.05 59.05,19.05 U1.6
SEGF
  Bottom 0.203: R7.P$2 33.66,28.58 34.93,27.3 41.27,27.3 48.26,20.32 48.26,13.97 48.9,13.34 74.93,13.34 U1.11
SEGG
  Top 0.203: U1.12 80.01,13.34 85.09,13.34 86.99,15.24 R19.P$2
SHUTDOWN  (via drill 0.61)
  Top 0.203: U3.1 9.38,13.48 R58.P$1 | ATTINY.2 33.66,12.07 v28.57,12.07 | R59.P$1 10.79,8.26 18.41,8.26 19.68,6.98 v23.49,6.98
  Bottom 0.203: R58.P$1 R59.P$1 | v28.57,12.07 23.81,7.3 v23.49,6.98
TINY_2
  Top 0.203: ATTINY.7 36.2,23.49 34.93,24.77 4.45,24.77 J2.1
TINY_4
  Top 0.203: J1.1 4.45,24.13 29.21,24.13 35.56,17.78 36.83,17.78 38.73,15.88 ATTINY.3
UB
  Top 0.305: Q24.3 107.31,44.45 107.31,50.48 105.09,52.71 85.72,52.71 J4.9
  Bottom 0.305: R24.P$1 111.44,33.97 111.44,40.32 Q24.3
VCC  (via drill 0.61)
  Top 0.203: U1.20 66.04,17.15 U1.7 66.04,12.7 64.77,11.43 58.42,11.43 R66.P$2 60.96,5.08 | R67.P$2 92.71,16.51 92.71,12.7 92.07,12.07 | 92.07,12.07 U2.2 | C8.1 94.61,9.53 92.07,12.07 | R63.P$1 34.29,5.71 34.93,5.08 | 34.93,5.08 29.84,5.08 29.21,5.71 R62.P$1 | 45.09,5.08 44.45,5.71 R65.P$1 | 34.93,5.08 40.01,5.08 | 40.01,5.08 45.09,5.08 | R64.P$1 39.37,5.71 40.01,5.08 | C8.1 88.27,1.91 85.09,5.08 81.91,5.08 C7.2 D1.C 73.27,5.08 60.96,5.08 | U3.6 14.93,20.01 v14.62,20.32 20.32,20.32 | 45.09,5.08 60.96,5.08 | U$10.IN+ 113.03,1.91 100.96,1.91 99.69,3.18 95.88,3.18 C8.1 | 20.32,20.32 21.59,19.05 R60.P$2 | C3.1 24.13,21.59 22.86,20.32 20.32,20.32
  Bottom 0.203: R67.P$2 R68.P$2 96.52,19.69 100.96,19.69 R69.P$2 | R62.P$1 31.11,8.89 31.11,19.69 ATTINY.8 C3.1 | v14.62,20.32 10.16,20.32 8.26,18.41 R58.P$2 5.71,14.61 5.71,5.71 6.99,4.45 C1.1
VIN
  Top 0.305: R29.P$2 Q2.1 6.99,41.27 8.89,39.37 | R31.P$2 Q4.1 15.88,40.64 17.14,39.37 | 8.89,39.37 17.14,39.37 | 17.14,39.37 26.04,39.37 | 26.04,39.37 34.93,39.37 | 34.93,39.37 43.82,39.37 | 43.82,39.37 52.71,39.37 | 52.71,39.37 61.59,39.37 | 61.59,39.37 70.48,39.37 | 70.48,39.37 79.38,39.37 | 79.38,39.37 88.27,39.37 | 88.27,39.37 97.16,39.37 | 97.16,39.37 106.05,39.37 | 106.05,39.37 114.93,39.37 | 114.93,39.37 120.02,39.37 Q28.1 R55.P$2 | R33.P$2 Q6.1 24.76,40.64 26.04,39.37 | R35.P$2 Q8.1 33.66,40.64 34.93,39.37 | R37.P$2 Q10.1 42.55,40.64 43.82,39.37 | R39.P$2 Q12.1 51.44,40.64 52.71,39.37 | R41.P$2 Q14.1 60.33,40.64 61.59,39.37 | R43.P$2 Q16.1 69.21,40.64 70.48,39.37 | R45.P$2 Q18.1 78.1,40.64 79.38,39.37 | R47.P$2 Q20.1 86.99,40.64 88.27,39.37 | R49.P$2 Q22.1 95.88,40.64 97.16,39.37 | R51.P$2 Q24.1 104.77,40.64 106.05,39.37 | R53.P$2 Q26.1 113.66,40.64 114.93,39.37 | 8.89,39.37 JP3.2

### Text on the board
Unrouted: This work is licensed under a Creative Commons Attribution-NonCommercial-ShareAlike 4.0 International License. / http://creativecommons.org/licenses/by-nc-sa/4.0/deed.en_US
tNames: FUTABA 5LT43 | F1 | F2 | G4 | D | E | F | A | G3 | CL1 | B | GC | C | G | G2 | UB | CL2 | G1 | LB | 47K | 47K | 2N3906 | GND | 25V | TINY | D2 | 4.7K | 10K | 2N3904 | VFD CLOCK | KEVIN RYE | 2017 | 3V OUT | D4 | ENABLE | ALARM | MINS | HOURS | SPEAKER | GND | 5V | V1.0 | PWR IN | GND | 5V IN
